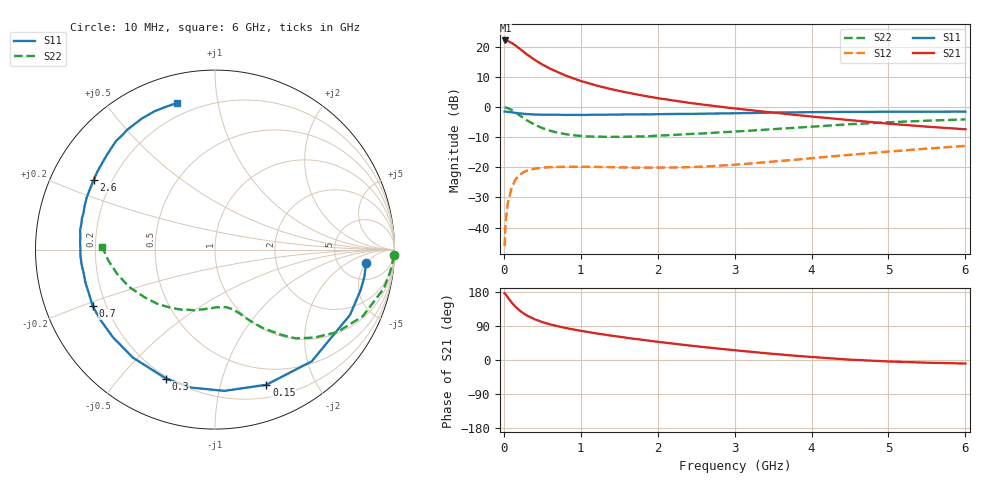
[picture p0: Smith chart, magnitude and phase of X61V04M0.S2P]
! SIEMENS Small Signal Semiconductors
! BFP193W
! Si NPN RF Bipolar Junction Transistor in SOT343
! VCE = 1 V  IC = 4 mA
! Common Emitter S-Parameters:  April 1994
# GHz  S  MA  R  50
!  f  S11  S21  S12  S22
! GHz  MAG  ANG  MAG  ANG  MAG  ANG  MAG  ANG
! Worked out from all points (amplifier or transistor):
!   40 points, 10 MHz to 6 GHz, reference 50 ohm
!   highest |S21| = 22.2 dB at 20 MHz (marker M1)
!   |S21| within 3 dB of that: start of sweep to 218.6 MHz
!   unconditionally stable (mu >= 1): 1.712 GHz to end of sweep
!   at 200 MHz: K = 0.13, MSG = 21.1 dB, |S12| = -22.6 dB
!   at 1.5 GHz: K = 0.89, MSG = 12.7 dB, |S12| = -20.0 dB
!   at 6 GHz: K = 1.03, MAG = 1.8 dB, |S12| = -12.9 dB
!   S11 on the Smith chart (normalised r, x): 10 MHz: 9, -5; 150 MHz: 0.33, -1.40; 300 MHz: 0.19, -0.67; 700 MHz: 0.15, -0.22; 2.6 GHz: 0.13, +0.26; 6 GHz: 0.13, +0.76
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0.01  0.8457 -5.1  12.8 176.3  0.0049 88.1  0.9957 -1.8
0.02  0.8457 -10.4  12.87 174.3  0.0102 85.1  0.9894 -5.4
0.05  0.8357 -25.8  12.61 165.6  0.0248 77.0  0.9656 -12.9
0.1  0.8234 -49.1  11.74 152.4  0.0455 65.0  0.9036 -24.2
0.15  0.8057 -69.2  10.67 140.7  0.0625 54.7  0.8222 -34.0
0.2  0.7888 -86.2  9.501 131.4  0.0738 46.9  0.7395 -41.5
0.25  0.7801 -99.7  8.48 123.9  0.0825 40.6  0.6702 -47.6
0.3  0.7689 -110.7  7.54 117.5  0.0882 35.8  0.6049 -51.9
0.4  0.756 -127.3  6.146 107.6  0.095 28.7  0.5124 -58.6
0.5  0.7496 -139.4  5.132 100.0  0.0988 24.3  0.4501 -63.1
0.6  0.7486 -148.3  4.383 94.1  0.1008 20.9  0.4071 -66.7
0.7  0.7509 -155.2  3.834 89.2  0.1017 18.8  0.3768 -69.3
0.9  0.7449 -165.8  3.027 80.7  0.1024 16.0  0.3425 -74.4
1.1  0.7478 -173.6  2.51 73.6  0.1021 14.7  0.3263 -78.9
1.3  0.7501 179.7  2.135 67.2  0.1013 14.3  0.3223 -83.7
1.6  0.7592 171.7  1.758 58.5  0.0999 15.5  0.3234 -90.4
2.2  0.7716 157.9  1.296 43.3  0.0996 20.9  0.3455 -104.5
2.6  0.7798 150.0  1.1 34.1  0.1031 26.0  0.3665 -114.0
3.2  0.7998 139.1  0.896 21.9  0.1158 32.4  0.4078 -127.6
4.5  0.8361 119.3  0.61 0.9  0.1618 37.1  0.5219 -156.5
5.5  0.8412 109.3  0.475 -7.1  0.2051 34.5  0.5967 -174.0
6  0.8442 104.7  0.43 -9.3  0.2275 32.3  0.6272 178.9
